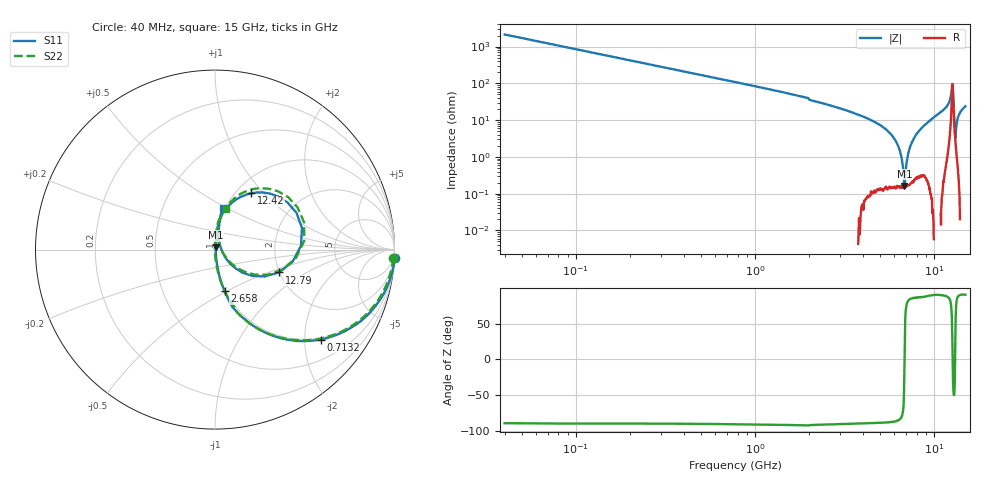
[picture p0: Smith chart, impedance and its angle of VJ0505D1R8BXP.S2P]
! VJ0505D1R8BXP
! MLCC placed on 25 mil thick microstrip substrate in series configuraton.
! DATE 06/29/2018  07:31
! CORRECTED  DATA
# GHz  S  MA  R  50.00
!  FREQ  S11M  S11A  S21M  S21A  S12M  S12A  S22M  S22A
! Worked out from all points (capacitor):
!   401 points, 40 MHz to 15 GHz, reference 50 ohm
!   read as one part in series: C = 1.86 pF near 114.8 MHz
!   lowest |Z| = 161 mohm at 6.847 GHz (marker M1)
!   series resonance near 6.855 GHz, so ESL is about 290 pH
!   S11 on the Smith chart (normalised r, x): 40 MHz: -2, -43; 713.2 MHz: 0.96, -2.38; 2.658 GHz: 0.99, -0.48; 12.42 GHz: 1.17, +0.85; 12.79 GHz: 1.99, -0.59; 15 GHz: 0.98, +0.48
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0.04  1.002 -2.7  0.04673 86.9  0.04744 87.7  0.9948 -2.7
0.2644  0.9597 -17.2  0.2965 72.9  0.2967 72.9  0.9519 -17.1
0.7132  0.7731 -40.4  0.6497 50.5  0.6501 50.6  0.7675 -40.2
1.4612  0.4952 -62.0  0.8861 30.0  0.8865 30.0  0.4945 -62.0
2.5458  0.2506 -76.4  0.9735 15.2  0.9739 15.3  0.2516 -76.0
2.658  0.236 -77.0  0.9761 14.4  0.9767 14.5  0.238 -76.8
5.0516  0.06082 -82.3  0.9964 4.7  0.9967 4.7  0.06012 -86.4
6.0614  0.01737 -76.3  0.9979 2.4  0.9981 2.4  0.01685 -92.1
6.2858  0.00944 -65.2  0.9978 1.9  0.9985 1.9  0.008796 -97.3
6.5102  0.003675 -1.4  0.9979 1.4  0.9983 1.4  0.001168 -162.5
6.8468  0.01237 75.4  0.9978 0.7  0.9982 0.7  0.0119 94.2
7.52  0.03635 84.5  0.9964 -0.7  0.997 -0.7  0.03622 89.7
10.0258  0.1284 83.3  0.9906 -6.2  0.9917 -6.2  0.1315 84.6
11.8584  0.2379 74.8  0.9614 -13.1  0.962 -13.0  0.2465 74.8
12.4194  0.3732 57.2  0.8571 -21.0  0.8574 -21.0  0.3884 59.2
12.5316  0.4363 45.8  0.7632 -23.9  0.7635 -23.9  0.4539 48.3
12.6812  0.4993 14.0  0.5255 -13.3  0.5257 -13.2  0.5191 17.0
12.7934  0.3786 -19.6  0.6488 12.0  0.6489 12.0  0.3929 -16.4
13.0926  0.04558 -20.6  0.9576 1.7  0.9582 1.8  0.04498 -19.6
13.1674  0.03405 27.8  0.9709 -0.2  0.9714 -0.2  0.03301 31.8
13.691  0.1292 80.5  0.9878 -6.9  0.9885 -6.8  0.1313 83.2
15  0.2344 78.7  0.9738 -13.3  0.9742 -13.3  0.2358 75.4
